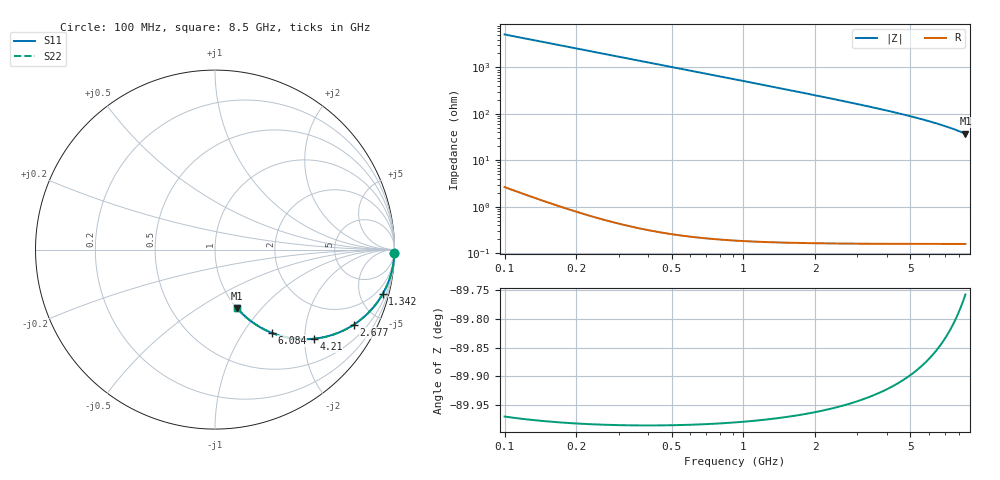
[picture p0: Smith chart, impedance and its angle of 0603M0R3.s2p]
! Created Wed Apr 18 11:48:50 2012
# hz S ma R 50
! 2 Port Network Data from SP1.SP block
! freq  magS11  angS11  magS21  angS21  magS12  angS12  magS22  angS22
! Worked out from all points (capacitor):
!   8401 points, 100 MHz to 8.5 GHz, reference 50 ohm
!   read as one part in series: C = 310 fF near 142 MHz
!   lowest |Z| = 37.3 ohm at 8.5 GHz (marker M1)
!   S11 on the Smith chart (normalised r, x): 100 MHz: open; 1.342 GHz: 1.00, -7.58; 2.677 GHz: 1.00, -3.69; 4.21 GHz: 1.00, -2.21; 6.084 GHz: 1.00, -1.36; 8.5 GHz: 1.00, -0.75
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1e8  0.9998 -1.1  0.01948 88.9  0.01948 88.9  0.9998 -1.1
1.24e8  0.9997 -1.4  0.02415 88.6  0.02415 88.6  0.9997 -1.4
1.92e8  0.9993 -2.1  0.03738 87.8  0.03738 87.8  0.9993 -2.1
2.66e8  0.9986 -3.0  0.05176 87.0  0.05176 87.0  0.9986 -3.0
3.7e8  0.9974 -4.1  0.07193 85.9  0.07193 85.9  0.9974 -4.1
4.99e8  0.9953 -5.6  0.09686 84.4  0.09686 84.4  0.9953 -5.6
6.6e8  0.9918 -7.3  0.1278 82.6  0.1278 82.6  0.9918 -7.3
8.53e8  0.9863 -9.5  0.1645 80.5  0.1645 80.5  0.9863 -9.5
1.08e9  0.9782 -12.0  0.2071 78.0  0.2071 78.0  0.9782 -12.0
1.342e9  0.9668 -14.8  0.2551 75.2  0.2551 75.2  0.9668 -14.8
1.5e9  0.9588 -16.5  0.2835 73.5  0.2835 73.5  0.9588 -16.5
2.035e9  0.9266 -22.1  0.3755 67.9  0.3755 67.9  0.9266 -22.1
2.677e9  0.8789 -28.4  0.4763 61.5  0.4763 61.5  0.8789 -28.4
2.9e9  0.8605 -30.6  0.5086 59.4  0.5086 59.4  0.8605 -30.6
3.539e9  0.8041 -36.4  0.5935 53.5  0.5935 53.5  0.8041 -36.4
4.21e9  0.741 -42.1  0.6704 47.8  0.6704 47.8  0.741 -42.1
4.3e9  0.7324 -42.8  0.6798 47.1  0.6798 47.1  0.7324 -42.8
4.966e9  0.6681 -48.0  0.7429 41.9  0.7429 41.9  0.6681 -48.0
5.7e9  0.5974 -53.2  0.8007 36.7  0.8007 36.7  0.5974 -53.2
6.084e9  0.5611 -55.7  0.8265 34.1  0.8265 34.1  0.5611 -55.7
7.1e9  0.4681 -61.9  0.8823 27.9  0.8823 27.9  0.4681 -61.9
8.5e9  0.3493 -69.3  0.9355 20.4  0.9355 20.4  0.3493 -69.3
